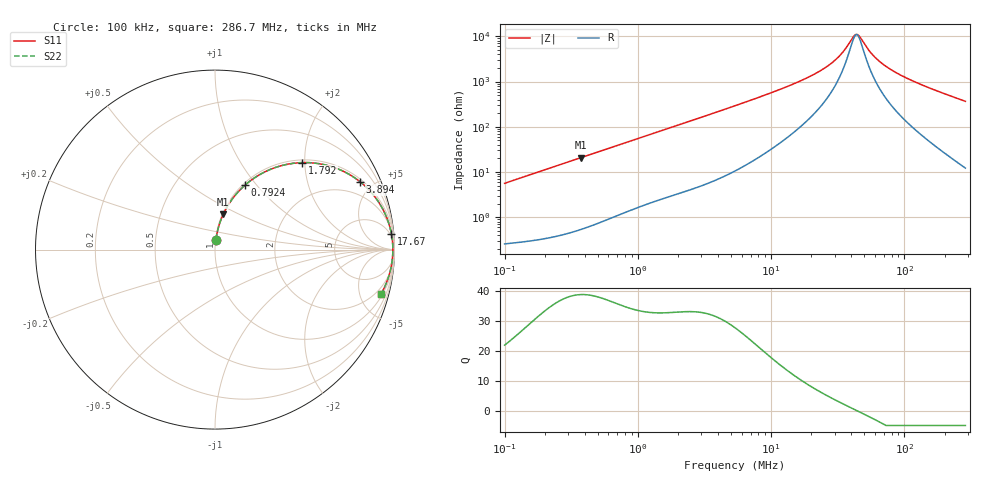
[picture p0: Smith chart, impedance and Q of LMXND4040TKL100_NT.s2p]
! LMXND4040TKL100_NT  S-PARAMETER MODEL  ( Standard Model )
! Model Generated by TAIYO YUDEN Corporation (https://www.yuden.co.jp/en/)
! Version 1.0
! TAIYO YUDEN Control No. 20250409
! Copyright(c) 2025 TAIYO YUDEN CO.,LTD. All Rights Reserved.
! Product Description (link to TY-COMPAS)
! https://ds.yuden.co.jp/TYCOMPAS/or/detail?pn=LMXND4040TKL100MNT&u=M
! Products Name : Inductors
! Characteristics :
!  Inductance : 10 [uH] , SRF(min) : 25 [MHz] , DC Resistance(max) : 0.18 [Ohm]
!  Rated Current : Saturation  1300 [mA] , Temp Rise  1500 [mA] (40 [degC])
!  Case Size : 4.0 x 4.0 / 0.157 x 0.157 [mm/inch] , Thickness : 1.8 / 0.071 [mm/inch]
!  (Conditions: Temperature = 25 [degC] , DC Bias Current = 0 [A])
! External Node Assignments :
!  1  o---GGG---o  2
! GND o---------o GND
! Frequency Range : 0.1MHz  -  286.687601MHz  [ 402 STEP ]
# MHz S RI R 50
! Freq[MHz].  S11 Real  S11 Imag  S21 Real  S21 Imag  S12 Real  S12 Imag  S22 Real  S22 Imag
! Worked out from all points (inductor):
!   401 points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, 100 kHz to 286.7 MHz, reference 50 ohm
!   read as one part in series: L = 8.92 uH near 104.1 kHz
!   highest Q = 38.7 at 371.9 kHz (marker M1), where L = 8.86 uH
!   self-resonance near 43.28 MHz
!   S11 on the Smith chart (normalised r, x): 100 kHz: 1.01, +0.11; 792.4 kHz: 1.03, +0.87; 1.792 MHz: 1.06, +1.95; 3.894 MHz: 1.13, +4.22; 17.67 MHz: 3, +22; 286.7 MHz: 1.24, -7.31
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0.1  0.00569 0.0558  0.9943 -0.0558  0.9943 -0.0558  0.00569 0.0558
0.37194  0.0458 0.1965  0.9542 -0.1965  0.9542 -0.1965  0.0458 0.1965
0.379416  0.0474 0.2  0.9526 -0.2  0.9526 -0.2  0.0474 0.2
0.792367  0.1674 0.3592  0.8326 -0.3592  0.8326 -0.3592  0.1674 0.3592
1.439567  0.3847 0.4715  0.6153 -0.4715  0.6153 -0.4715  0.3847 0.4715
1.791887  0.4871 0.4848  0.5129 -0.4848  0.5129 -0.4848  0.4871 0.4848
2.563859  0.6539 0.4608  0.3461 -0.4608  0.3461 -0.4608  0.6539 0.4608
3.894109  0.8089 0.3776  0.1911 -0.3776  0.1911 -0.3776  0.8089 0.3776
5.354322  0.8862 0.3  0.1138 -0.3  0.1138 -0.3  0.8862 0.3
10.53378  0.9639 0.1592  0.0361 -0.1592  0.0361 -0.1592  0.9639 0.1592
17.67322  0.9832 0.0861  0.0168 -0.0861  0.0168 -0.0861  0.9832 0.0861
20.31517  0.9858 0.0704  0.0142 -0.0704  0.0142 -0.0704  0.9858 0.0704
25.79543  0.9888 0.0462  0.0112 -0.0462  0.0112 -0.0462  0.9888 0.0462
30.85563  0.9901 0.0298  0.00994 -0.0298  0.00994 -0.0298  0.9901 0.0298
35.46819  0.9907 0.0177  0.00933 -0.0177  0.00933 -0.0177  0.9907 0.0177
41.58984  0.991 0.00421  0.00901 -0.00421  0.00901 -0.00421  0.991 0.00421
43.27871  0.991 0.000873  0.00899 -0.000873  0.00899 -0.000873  0.991 0.000873
45.94147  0.991 -0.00414  0.009 0.00414  0.009 0.00414  0.991 -0.00414
59.50735  0.9903 -0.0262  0.00966 0.0262  0.00966 0.0262  0.9903 -0.0262
77.07906  0.9885 -0.05  0.0115 0.05  0.0115 0.05  0.9885 -0.05
129.3207  0.979 -0.1085  0.021 0.1085  0.021 0.1085  0.979 -0.1085
286.6876  0.9232 -0.2501  0.0768 0.2501  0.0768 0.2501  0.9232 -0.2501
